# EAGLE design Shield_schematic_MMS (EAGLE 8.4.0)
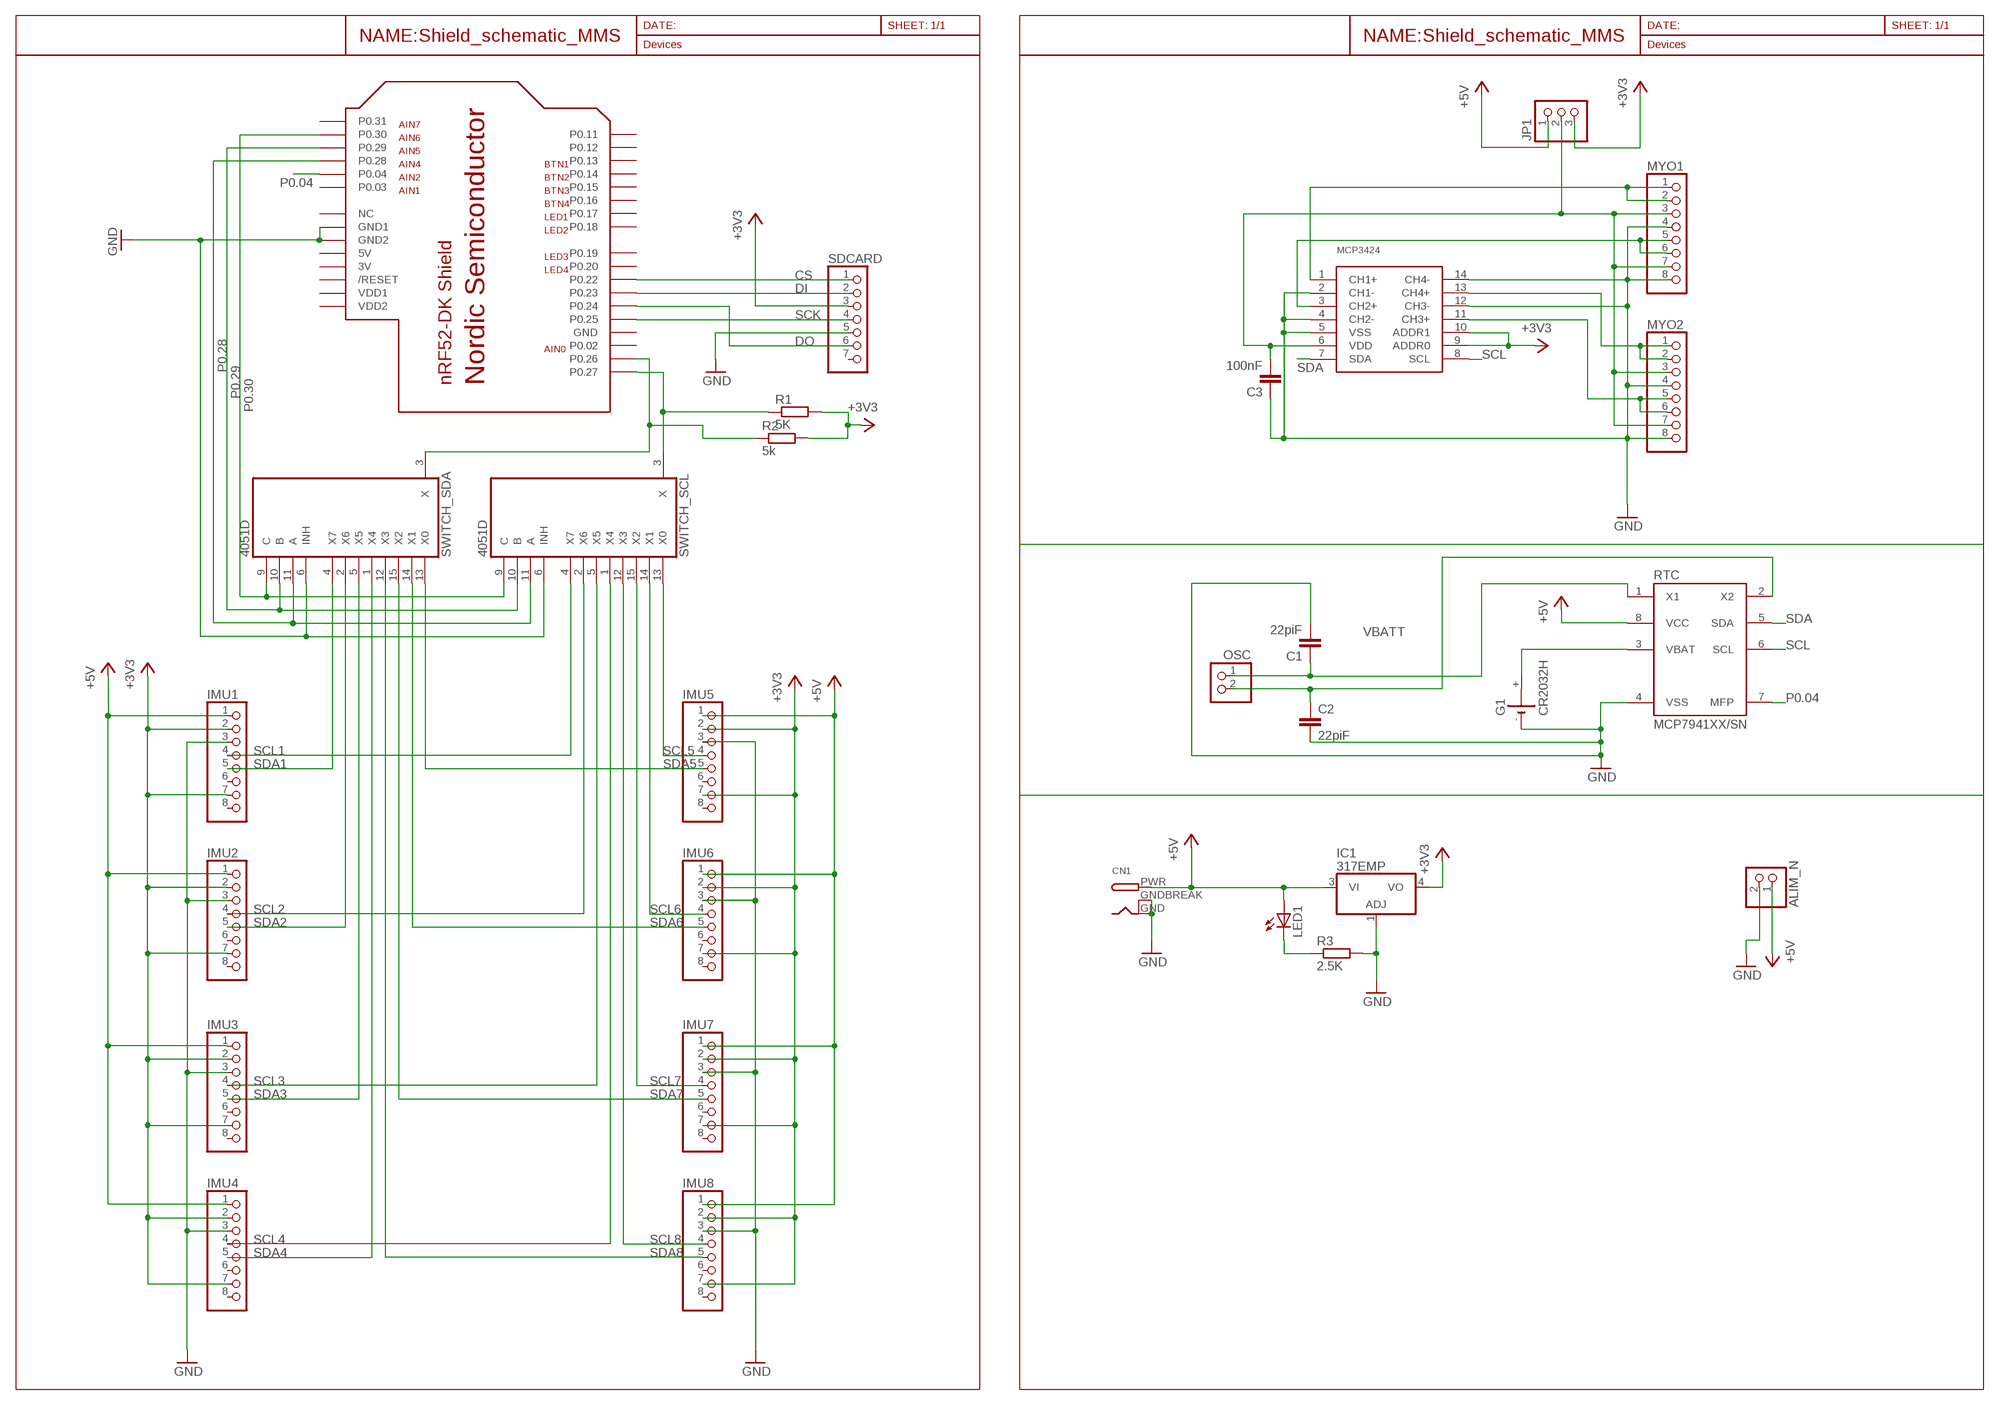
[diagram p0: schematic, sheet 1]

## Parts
ALIM_N  PINHD-1X2  [1X02]
C1  22piF  C2.5/2  [C2.5-2]
C2  22piF  C2.5/2  [C2.5-2]
C3  100nF  C2.5/2  [C2.5-2]
CN1  DCBARRELPTH  [DCJACK_2MM_PTH]
G1  CR2032H  [CR2032H]
IC1  317EMP  [SOT223]
IMU1  PINHD-1X8  [1X08]
IMU2  PINHD-1X8  [1X08]
IMU3  PINHD-1X8  [1X08]
IMU4  PINHD-1X8  [1X08]
IMU5  PINHD-1X8  [1X08]
IMU6  PINHD-1X8  [1X08]
IMU7  PINHD-1X8  [1X08]
IMU8  PINHD-1X8  [1X08]
JP1  PINHD-1X3  [1X03]
LED1  LEDCHIPLED_1206  [CHIPLED_1206]
MYO1  PINHD-1X8  [1X08]
MYO2  PINHD-1X8  [1X08]
OSC  PINHD-1X2  [1X02]
R1  5K  R-EU_M1206  [M1206]
R2  5k  R-EU_M1206  [M1206]
R3  2.5K  R-EU_M1206  [M1206]
RTC  MCP7941XX/SN  [SO8]
SDCARD  PINHD-1X7  [1X07]
SWITCH_SCL  4051D  [SO16]
SWITCH_SDA  4051D  [SO16]
U$2  NRF52-SHIELD-NOTEXT  [NRF52-SHIELD]
U$3  MCP3424  [SO14]

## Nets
+3V3: IC1.4(VO) IMU1.2 IMU1.7 IMU2.2 IMU2.7 IMU3.2 IMU3.7 IMU4.2 IMU4.7 IMU5.2 IMU5.7 IMU6.2 IMU6.7 IMU7.2 IMU7.7 IMU8.2 IMU8.7 JP1.3 R1.2 R2.2 SDCARD.3 U$3.9(ADDR0) U$3.10(ADDR1)
+5V: ALIM_N.1 CN1.PWR IC1.3(VI) IMU1.1 IMU2.1 IMU3.1 IMU4.1 IMU5.1 IMU6.1 IMU7.1 IMU8.1 JP1.1 LED1.A RTC.8(VCC)
CH1: MYO1.1 MYO1.2 U$3.1(CH1+)
CH2: MYO1.5 MYO1.6 U$3.3(CH2+)
CH3: MYO2.5 MYO2.6 U$3.11(CH3+)
CH4: MYO2.1 MYO2.2 U$3.13(CH4+)
CS: SDCARD.1 U$2.P22(P0.22)
DI: SDCARD.2 U$2.P23(P0.23)
DO: SDCARD.6 U$2.P24(P0.24)
GND: ALIM_N.2 C1.2 C2.2 C3.1 CN1.GND CN1.GNDBREAK G1.- IC1.1(ADJ) IMU1.3 IMU2.3 IMU3.3 IMU4.3 IMU5.3 IMU6.3 IMU7.3 IMU8.3 MYO1.4 MYO1.8 MYO2.4 MYO2.8 R3.2 RTC.4(VSS) SDCARD.5 SWITCH_SCL.6(INH) SWITCH_SDA.6(INH) U$2.GND1 U$2.GND2 U$3.2(CH1-) U$3.4(CH2-) U$3.5(VSS) U$3.12(CH3-) U$3.14(CH4-)
N$12: LED1.C R3.1
P0.04: RTC.7(MFP) U$2.P04(P0.04)
P0.28: SWITCH_SCL.11(A) SWITCH_SDA.11(A) U$2.P28(P0.28)
P0.29: SWITCH_SCL.10(B) SWITCH_SDA.10(B) U$2.P29(P0.29)
P0.30: SWITCH_SCL.9(C) SWITCH_SDA.9(C) U$2.P30(P0.30)
SCK: SDCARD.4 U$2.P25(P0.25)
SCL: R1.1 RTC.6(SCL) SWITCH_SCL.3(X) U$2.P27(P0.27) U$3.8(SCL)
SCL1: IMU1.4 SWITCH_SCL.4(X7)
SCL2: IMU2.4 SWITCH_SCL.2(X6)
SCL3: IMU3.4 SWITCH_SCL.5(X5)
SCL4: IMU4.4 SWITCH_SCL.1(X4)
SCL5: IMU5.4 SWITCH_SCL.13(X0)
SCL6: IMU6.4 SWITCH_SCL.14(X1)
SCL7: IMU7.4 SWITCH_SCL.15(X2)
SCL8: IMU8.4 SWITCH_SCL.12(X3)
SDA: R2.1 RTC.5(SDA) SWITCH_SDA.3(X) U$2.P26(P0.26) U$3.7(SDA)
SDA1: IMU1.5 SWITCH_SDA.4(X7)
SDA2: IMU2.5 SWITCH_SDA.2(X6)
SDA3: IMU3.5 SWITCH_SDA.5(X5)
SDA4: IMU4.5 SWITCH_SDA.1(X4)
SDA5: IMU5.5 SWITCH_SDA.13(X0)
SDA6: IMU6.5 SWITCH_SDA.14(X1)
SDA7: IMU7.5 SWITCH_SDA.15(X2)
SDA8: IMU8.5 SWITCH_SDA.12(X3)
VBATT: G1.+ RTC.3(VBAT)
VDD: C3.2 JP1.2 MYO1.3 MYO1.7 MYO2.3 MYO2.7 U$3.6(VDD)
X1: C1.1 OSC.1 RTC.1(X1)
X2: C2.1 OSC.2 RTC.2(X2)
Unconnected: G1.+@1(+) IMU1.6 IMU1.8 IMU2.6 IMU2.8 IMU3.6 IMU3.8 IMU4.6 IMU4.8 IMU5.6 IMU5.8 IMU6.6 IMU6.8 IMU7.6 IMU7.8 IMU8.6 IMU8.8 SDCARD.7 U$2.NC U$2.P02(P0.02) U$2.P03(P0.03) U$2.P11(P0.11) U$2.P12(P0.12) U$2.P13(P0.13) U$2.P14(P0.14) U$2.P15(P0.15) U$2.P16(P0.16) U$2.P17(P0.17) U$2.P18(P0.18) U$2.P19(P0.19) U$2.P20(P0.20) U$2.P31(P0.31) U$2.RESET(/RESET)

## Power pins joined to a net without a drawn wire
3V: U$2.3V
5V: U$2.5V
GND: SWITCH_SCL.8(GND) SWITCH_SDA.8(GND) U$2.GND
VCC: SWITCH_SCL.16(VCC) SWITCH_SDA.16(VCC)
VDD1: U$2.VDD2(VDD1)
VDD2: U$2.VDD1(VDD2)
VEE: SWITCH_SCL.7(VEE) SWITCH_SDA.7(VEE)

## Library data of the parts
ALIM_N OSC = pinhead:PINHD-1X2: PIN HEADER
C1-C3 = capacitor-wima:C: CAPACITOR
CN1 = adafruit:DCBARREL: 2.0mm DC Barrel Jack DCJACK_2MM_PTH - Through Hole Jack (4UConnector: 05537)
G1 = battery:CR2032H: LI BATTERY Varta
IC1 = linear:*317: Positive VOLTAGE REGULATOR
IMU1-IMU8 MYO1 MYO2 = pinhead:PINHD-1X8: PIN HEADER
JP1 = pinhead:PINHD-1X3: PIN HEADER
LED1 = adafruit:LED: LED
R1-R3 = resistor:R-EU_: RESISTOR, European symbol
RTC = _hhn_MCP7941X:MCP7941*?: Microchip MCP79410 / MCP79411 / MCP79412 I²C Real Time CLock/Calendar with Unique ID Rev. 5.0.0 as of 2013-10-23, for EAGLE 5+ Changelog 5.0.0 (initial) MCP79410XI/YY X: Unique ID 0: blank 1: EUI-48 2: EUI-96 I: Temperature Range (Industrial) /YY: Package /MS: MSOP8_.65 (8-Lead Micro Small Outline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
SDCARD = pinhead:PINHD-1X7: PIN HEADER
SWITCH_SCL SWITCH_SDA = 40xx:4051: 8-channel ANALOG MULTIPLEXER
U$2 = nrf52-shield_modif:NRF52-SHIELD: nRF5 devkit shield
U$3 = mcp3424:MCP3424

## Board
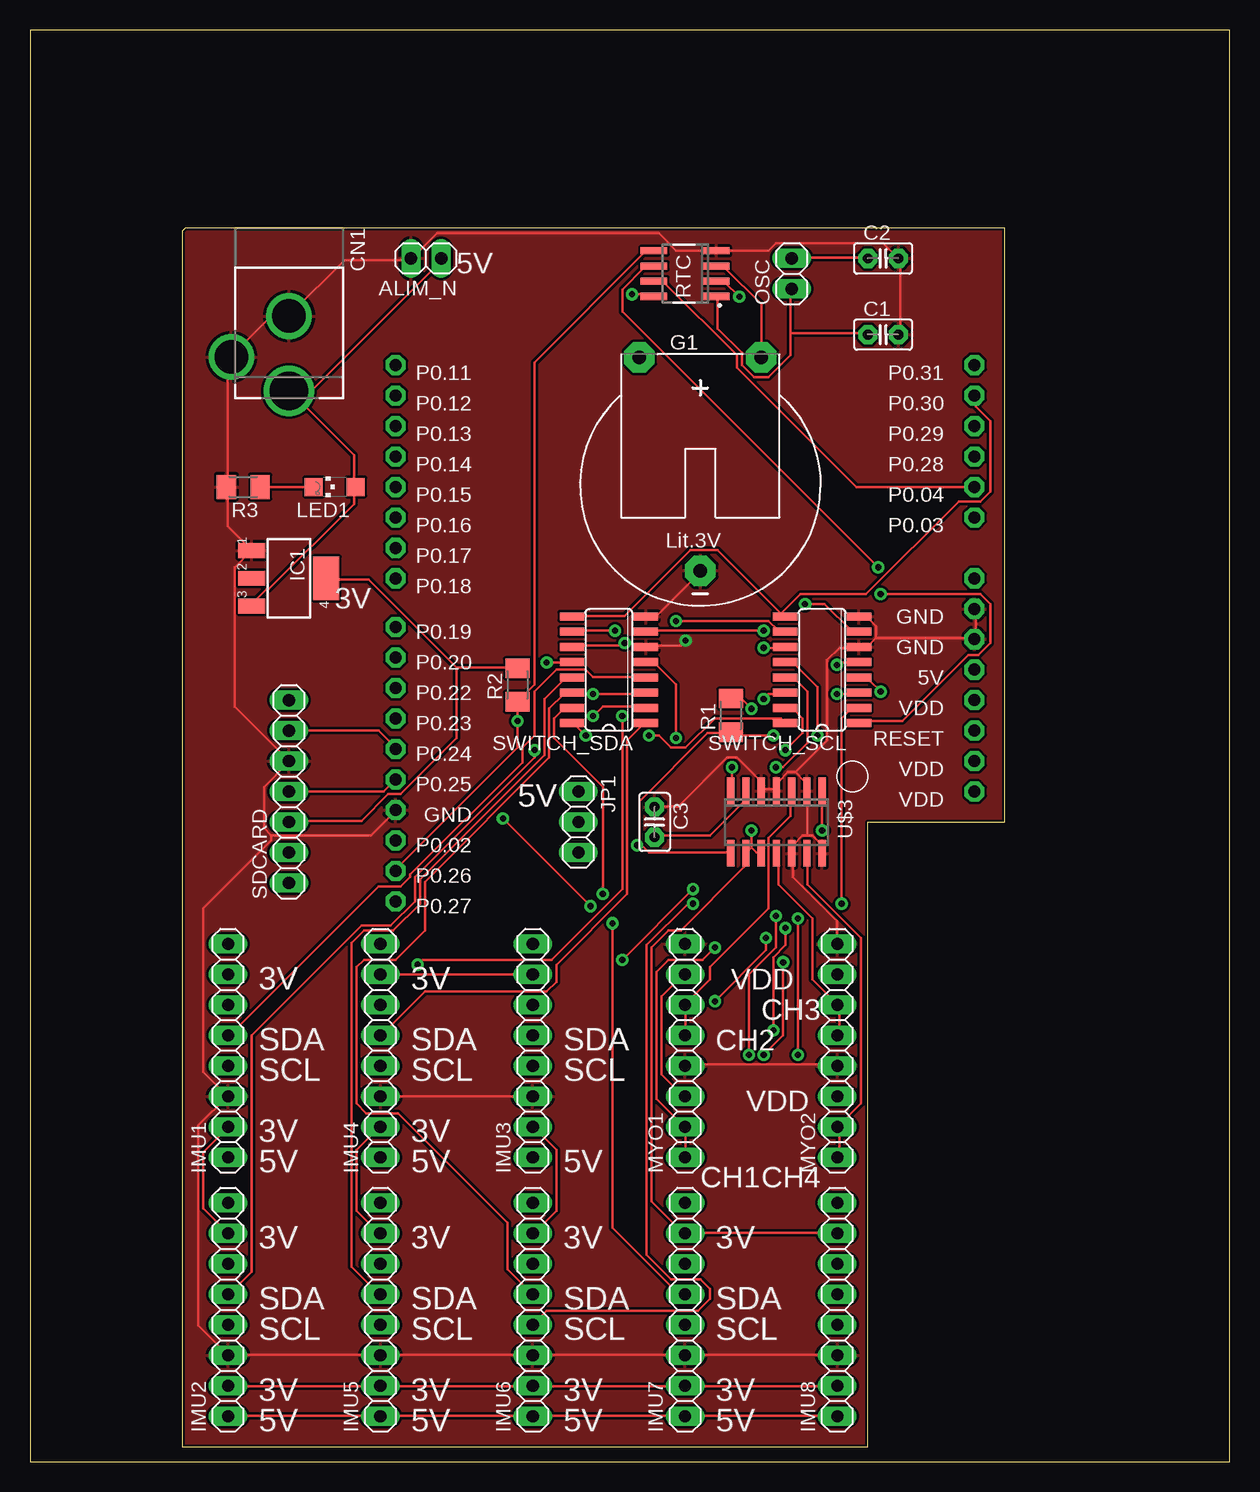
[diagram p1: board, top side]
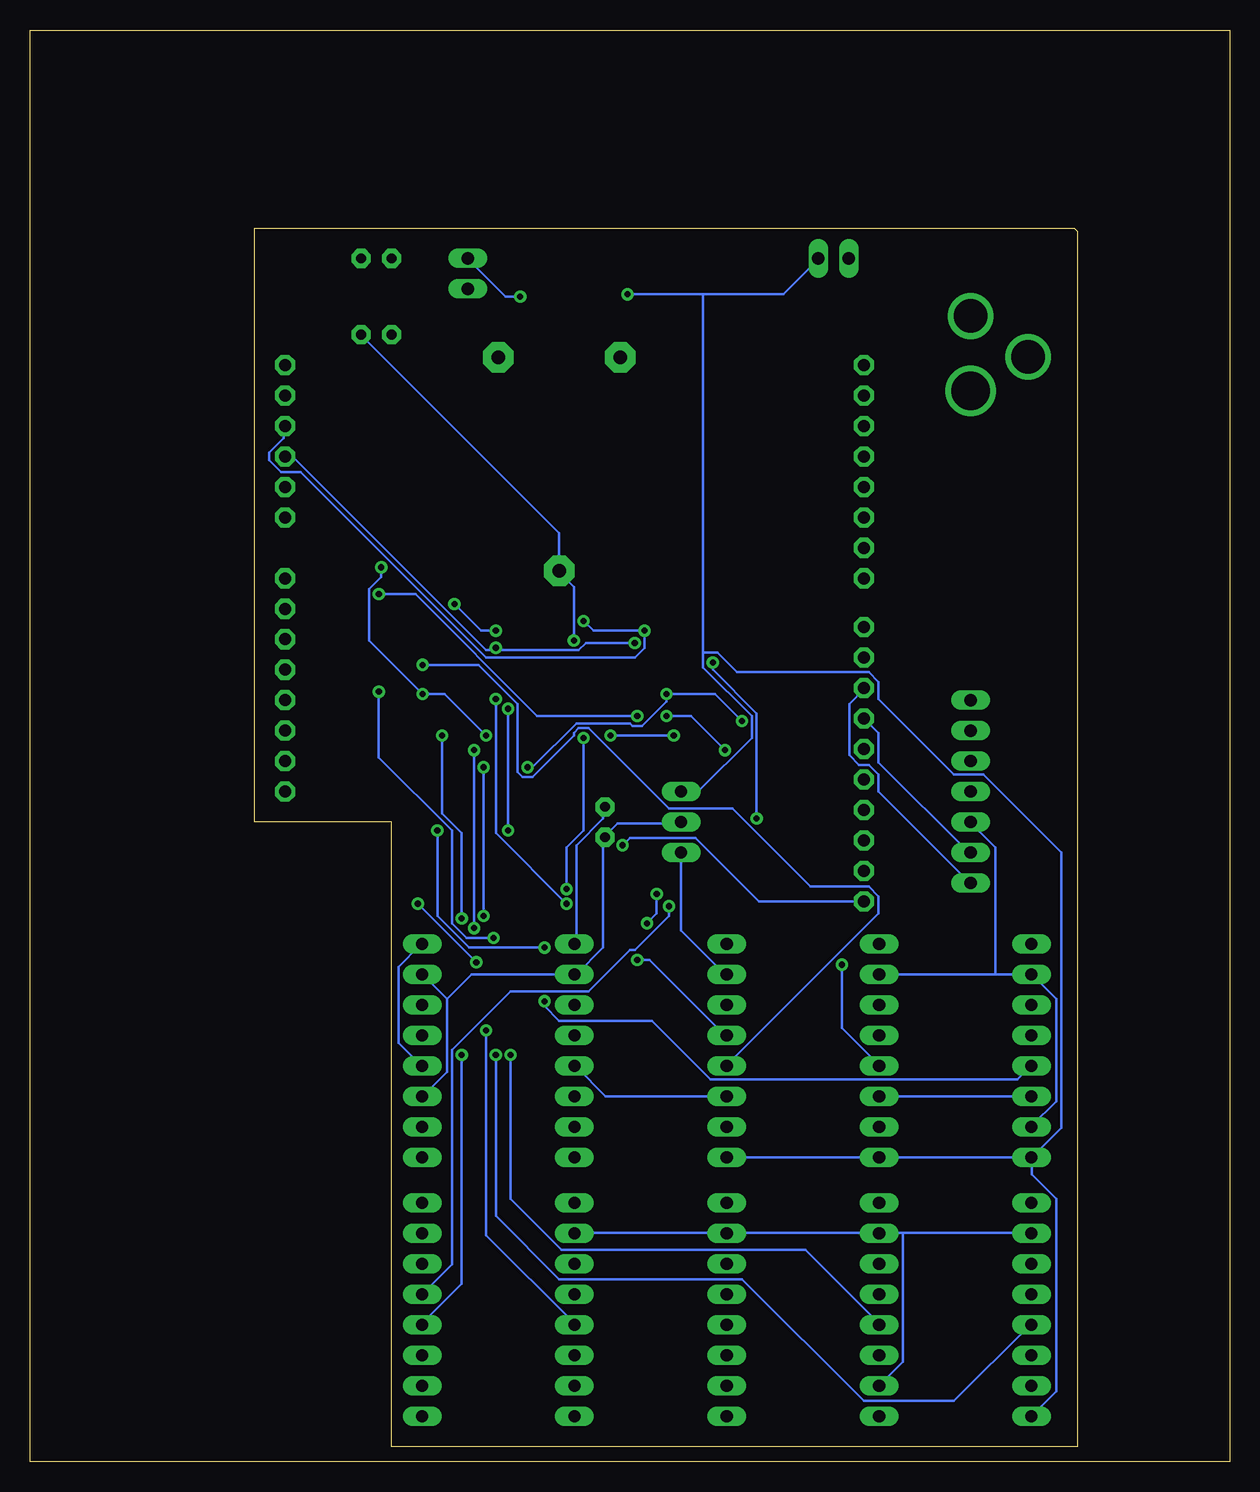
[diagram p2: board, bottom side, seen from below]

Size 100 x 119.37 mm. Coordinates in mm from the lower left corner, seen from the top.
Outline: 0,0 100,0 100,119.37 0,119.37 0,0
Copper layers (1*16): Top 0.035mm / dielectric 1.5mm / Bottom 0.035mm
Design rules "SparkFun": minimum track width 8mil, minimum drill 20mil, track to track 8mil, track to pad 8mil, pad to pad 8mil, via to via 8mil, smd to smd 8mil, copper to edge 8mil, drill to drill 8mil, minimum pad ring 12mil, minimum via ring 10mil, stop-mask expansion 4mil, vias tented up to drill 20mil, thermal gap 10mil

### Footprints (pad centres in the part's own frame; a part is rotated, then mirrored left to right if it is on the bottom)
1X02 = drill 1.016 long: 1 -1.27,0; 2 1.27,0
C2.5-2 = drill 0.813 pad 1.6 octagon: 1 -1.27,0; 2 1.27,0
DCJACK_2MM_PTH = drill 2.8: GND 0,7.35; GNDBREAK 4.8,10.75 | drill 3.2: PWR 0,13.6
CR2032H = drill 1.118 pad 2.54 octagon: + 5.08,10.795; +@1 -5.08,10.795; - 0,-6.985
SOT223 = smd 1.219 x 2.235: 1 -2.311,-3.099; 2 0,-3.099; 3 2.311,-3.099 | smd 3.6 x 2.2: 4 0,3.099
1X08 = drill 1.016 long: 1 -8.89,0; 2 -6.35,0; 3 -3.81,0; 4 -1.27,0; 5 1.27,0; 6 3.81,0; 7 6.35,0; 8 8.89,0
1X03 = drill 1.016 long: 1 -2.54,0; 2 0,0; 3 2.54,0
CHIPLED_1206 = smd 1.5 x 1.5: A 0,-1.75; C 0,1.75
M1206 = smd 1.6 x 2: 1 -1.4,0; 2 1.4,0
SO8 = smd 0.6 x 2.2: 1 -1.905,-2.6; 2 -0.635,-2.6; 3 0.635,-2.6; 4 1.905,-2.6; 5 1.905,2.6; 6 0.635,2.6; 7 -0.635,2.6; 8 -1.905,2.6
1X07 = drill 1.016 long: 1 -7.62,0; 2 -5.08,0; 3 -2.54,0; 4 0,0; 5 2.54,0; 6 5.08,0; 7 7.62,0
SO16 = smd 0.66 x 2.032: 1 -4.445,-3.073; 2 -3.175,-3.073; 3 -1.905,-3.073; 4 -0.635,-3.073; 5 0.635,-3.073; 6 1.905,-3.073; 7 3.175,-3.073; 8 4.445,-3.073; 9 4.445,3.073; 10 3.175,3.073; 11 1.905,3.073; 12 0.635,3.073; 13 -0.635,3.073; 14 -1.905,3.073; 15 -3.175,3.073; 16 -4.445,3.073
NRF52-SHIELD = drill 1 pad 1.676 octagon: 3V 62.23,1.27; 5V 64.77,1.27; GND 53.086,49.53; GND1 69.85,1.27; GND2 67.31,1.27; NC 72.39,1.27; P02 50.546,49.53; P03 77.47,1.27; P04 80.01,1.27; P11 90.17,49.53; P12 87.63,49.53; P13 85.09,49.53; P14 82.55,49.53; P15 80.01,49.53; P16 77.47,49.53; P17 74.93,49.53; P18 72.39,49.53; P19 68.326,49.53; P20 65.786,49.53; P22 63.246,49.53; P23 60.706,49.53; P24 58.166,49.53; P25 55.626,49.53; P26 48.006,49.53; P27 45.466,49.53; P28 82.55,1.27; P29 85.09,1.27; P30 87.63,1.27; P31 90.17,1.27; RESET 59.69,1.27; VDD1 57.15,1.27; VDD2 54.61,1.27
SO14 = smd 0.6 x 2.2: 1 -3.81,-2.6; 2 -2.54,-2.6; 3 -1.27,-2.6; 4 0,-2.6; 5 1.27,-2.6; 6 2.54,-2.6; 7 3.81,-2.6; 8 3.81,2.6; 9 2.54,2.6; 10 1.27,2.6; 11 0,2.6; 12 -1.27,2.6; 13 -2.54,2.6; 14 -3.81,2.6

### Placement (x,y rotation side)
ALIM_N  33.02,100.33 180 top
C1  71.12,93.98 0 top
C2  71.12,100.33 0 top
C3  52.07,53.34 270 top
CN1  21.59,102.87 180 top
G1  55.88,81.28 0 top
IC1  21.59,73.66 270 top
IMU1  16.51,34.29 90 top
IMU2  16.51,12.7 90 top
IMU3  41.91,34.29 90 top
IMU4  29.21,34.29 90 top
IMU5  29.21,12.7 90 top
IMU6  41.91,12.7 90 top
IMU7  54.61,12.7 90 top
IMU8  67.31,12.7 90 top
JP1  45.72,53.34 270 top
LED1  25.4,81.28 90 top
MYO1  54.61,34.29 90 top
MYO2  67.31,34.29 90 top
OSC  63.5,99.06 90 top
R1  58.42,62.23 90 top
R2  40.64,64.77 90 top
R3  17.78,81.28 180 top
RTC  54.61,99.06 90 top
SDCARD  21.59,55.88 90 top
SWITCH_SCL  66.04,66.04 90 top
SWITCH_SDA  48.26,66.04 90 top
U$2  80.01,1.27 90 top
U$3  62.23,53.34 180 top

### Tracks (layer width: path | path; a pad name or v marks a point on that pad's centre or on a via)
+3V3  (via drill 0.51)
  Top 0.203: 35.56,66.24 40.64,66.24 R2.2 | 35.56,66.24 28.25,73.56 24.79,73.56 IC1.4 | IMU4.7 IMU3.7 | 35.56,66.24 35.56,60.35 30.89,55.68 29.87,55.68 27.64,53.44 21.74,53.44 SDCARD.3 | IMU2.2 16.66,6.3 29.06,6.3 IMU5.2 29.26,6.3 41.86,6.3 IMU6.2 42.06,6.3 54.46,6.3 IMU7.2 54.66,6.3 67.26,6.3 IMU8.2 | IMU2.7 14.43,21.13 14.43,25.81 16.46,27.84 IMU1.2 | IMU5.7 29.06,19.1 27.23,20.93 27.23,26.01 29.06,27.84 IMU4.2 | v60.15,62.79 59.33,63.6 58.52,63.6 R1.2 | 60.15,51.21 v60.15,52.63 | 60.15,51.21 59.74,50.8 U$3.9 59.54,50.6 59.54,49.58 54.25,44.3 53.24,44.3 51.82,42.88 51.82,21.74 54.46,19.1 IMU7.7 54.66,19.1 67.26,19.1 IMU8.7 | 60.15,51.21 60.55,50.8 60.96,50.8 U$3.10 | IMU6.7 42.06,19.1 43.89,20.93 43.89,26.01 42.06,27.84 IMU3.2
  Bottom 0.203: JP1.3 45.72,44.3 42.06,40.64 IMU3.7 | IMU4.7 19.51,40.64 | 19.51,40.64 IMU1.7 16.46,40.64 14.43,38.61 14.43,30.07 16.46,28.04 IMU1.2 | 19.51,40.64 19.51,51.21 21.54,53.24 SDCARD.3 | 27.23,19.1 29.06,19.1 IMU5.7 29.26,19.1 41.86,19.1 IMU6.7 42.06,19.1 54.46,19.1 IMU7.7 | 27.23,19.1 16.66,19.1 IMU2.7 | v60.15,52.63 v60.15,62.79 | IMU5.2 27.23,8.33 27.23,19.1
+5V  (via drill 0.51)
  Top 0.203: IMU2.1 16.66,3.86 29.06,3.86 IMU5.1 29.26,3.86 41.86,3.86 IMU6.1 42.06,3.86 54.46,3.86 IMU7.1 54.66,3.86 67.26,3.86 IMU8.1 | 27.03,81.28 27.03,83.92 22.55,88.39 | 22.55,88.39 21.74,89.2 CN1.PWR 22.55,88.39 | 27.03,81.28 27.03,79.86 19.91,72.75 19.71,72.75 18.49,71.53 IC1.3 | 27.03,81.28 LED1.A | v50.19,97.33 51.82,97.33 RTC.8 | 22.55,88.39 34.34,100.18 ALIM_N.1
  Bottom 0.203: IMU3.1 IMU4.1 IMU1.1 16.46,25.4 | 16.46,25.4 16.46,23.98 14.43,21.95 14.43,5.89 IMU2.1 | 43.89,97.33 37.19,97.33 34.34,100.18 ALIM_N.1 | 43.89,97.33 v50.19,97.33 | JP1.1 44.3,55.88 39.83,60.35 39.83,62.18 43.89,66.24 43.89,67.46 | 43.89,97.33 43.89,67.46 | 16.46,25.4 14.02,27.84 14.02,50.8 20.52,57.3 22.96,57.3 29.26,63.6 29.26,65.02 30.07,65.84 41.05,65.84 42.67,67.46 43.89,67.46
CH1  (via drill 0.51)
  Top 0.203: v66.04,52.63 U$3.1 | v57.1,42.88 56.08,41.86 53.24,41.86 52.22,40.84 52.22,30.28 54.46,28.04 MYO1.2 54.66,27.84 54.66,25.4 MYO1.1
  Bottom 0.203: v66.04,52.63 66.04,45.52 63.4,42.88 v57.1,42.88
CH2
  Top 0.203: U$3.3 63.4,55.88 63.4,53.85 61.57,52.02 61.57,46.13 56.69,41.25 56.69,40.23 54.66,38.2 MYO1.6 54.66,38 54.66,35.56 MYO1.5
CH3
  Top 0.203: U$3.11 62.38,50.6 62.38,48.16 65.23,45.31 65.23,40.23 67.26,38.2 MYO2.6 67.46,38 67.46,35.56 MYO2.5
CH4
  Top 0.203: U$3.13 64.82,50.6 64.82,48.16 69.29,43.69 69.29,29.87 67.46,28.04 MYO2.2 67.46,27.84 67.46,25.4 MYO2.1
CS
  Bottom 0.203: SDCARD.1 21.74,48.36 29.26,55.88 29.26,57.3 30.07,58.12 30.89,58.12 31.7,58.93 31.7,63.2 30.48,64.41 U$2.P22
DI
  Bottom 0.203: U$2.P23 29.26,60.76 29.26,58.32 21.74,50.8 SDCARD.2
DO
  Top 0.203: SDCARD.6 29.06,60.96 30.48,59.54 U$2.P24
GND  (via drill 0.51)
  Top 0.203: v54.66,68.48 54.25,68.07 51.41,68.07 SWITCH_SDA.6 | SWITCH_SDA.8 51.41,70.51 52.22,70.51 55.88,74.17 G1.- | C1.2 72.54,94.08 72.54,100.18 C2.2 71.12,101.6 62.18,101.6 61.57,100.99 57.3,100.99 RTC.4 57.1,100.99 53.85,100.99 52.43,102.41 33.93,102.41 31.9,100.38 ALIM_N.2 31.7,100.18 26.21,100.18 21.74,95.71 CN1.GND 21.54,95.5 20.12,95.5 16.87,92.25 CN1.GNDBREAK 16.66,92.05 16.46,91.85 16.46,81.28 | 20.12,52.22 19.51,52.83 19.51,56.29 21.54,58.32 SDCARD.5 21.54,58.52 17.07,62.99 17.07,74.57 18.49,76 | 20.12,52.22 28.45,52.22 30.48,54.25 U$2.GND | 16.46,81.28 16.46,78.03 18.49,76 | 16.46,81.28 R3.2 | 18.49,76 IC1.1 | IMU8.3 67.26,8.94 54.66,8.94 IMU7.3 54.46,8.94 42.06,8.94 IMU6.3 41.86,8.94 29.26,8.94 IMU5.3 29.06,8.94 16.66,8.94 IMU2.3 14.02,11.38 14.02,28.04 16.46,30.48 | IMU4.3 IMU3.3 | MYO1.4 54.66,33.12 67.26,33.12 MYO2.4 | 70.51,68.68 69.9,68.07 69.29,68.07 SWITCH_SCL.6 69.09,67.87 67.46,67.87 66.45,66.85 66.45,60.15 63.8,57.51 | 70.51,68.68 70.51,69.7 69.9,70.31 69.29,70.31 SWITCH_SCL.8 | 70.51,68.68 78.64,68.68 U$2.GND2 78.84,68.68 78.84,71.12 U$2.GND1 | 60.96,56.08 62.18,56.08 U$3.4 62.38,56.08 62.38,56.69 63.2,57.51 63.8,57.51 | 64.82,52.22 65.23,52.22 66.04,51.41 U$3.14 | 64.82,52.22 64.41,52.22 63.6,51.41 63.6,50.8 U$3.12 63.6,50.6 63.6,48.77 67.26,45.11 67.26,43.28 MYO2.8 | 64.82,52.22 64.82,55.88 U$3.2 64.62,56.08 64.62,56.69 63.8,57.51 | 60.96,56.08 60.96,56.69 58.93,58.73 58.12,58.73 54.05,54.66 52.22,54.66 C3.1 | 60.96,56.08 U$3.5 | 20.12,52.22 20.12,51.82 14.43,46.13 14.43,32.51 16.46,30.48 | 16.46,30.48 IMU1.3
  Bottom 0.203: v54.66,68.48 54.66,72.95 55.88,74.17 G1.- 55.88,77.42 72.34,93.88 C1.2 | IMU4.3 IMU1.3 | C3.1 52.22,54.46 52.22,53.65 54.46,51.41 54.46,43.28 MYO1.8 | MYO2.4 67.46,33.12 69.29,34.95 69.29,41.25 67.46,43.08 MYO2.8 | IMU3.3 52.02,30.48 54.46,32.92 MYO1.4
  pour Top: 12.7,102.87 81.28,102.87 81.28,53.34 69.85,53.34 69.85,1.27 12.7,1.27
N$12
  Top 0.203: R3.1 LED1.C
P0.04
  Top 0.203: U$2.P04 68.89,81.28 58.93,91.24 58.93,92.25 52.83,98.35 52.02,98.35 RTC.7
P0.28  (via drill 0.51)
  Top 0.203: v49.58,68.28 49.38,68.07 45.31,68.07 SWITCH_SDA.11 | v61.16,67.87 62.79,67.87 SWITCH_SCL.11
  Bottom 0.203: v49.58,68.28 53.65,68.28 54.25,67.67 61.16,67.67 | 61.16,67.67 61.98,67.67 78.03,83.72 78.64,83.72 U$2.P28 | 61.16,67.67 v61.16,67.87
P0.29  (via drill 0.51)
  Top 0.203: v48.77,69.29 45.31,69.29 SWITCH_SDA.10 | v53.85,70.1 61.57,70.1 62.38,69.29 62.79,69.29 SWITCH_SCL.10
  Bottom 0.203: v53.85,70.1 53.03,69.29 v48.77,69.29 48.77,67.87 49.58,67.06 61.98,67.06 77.42,82.5 79.05,82.5 80.06,83.52 80.06,84.12 78.84,85.34 78.84,86.36 U$2.P29
P0.30
  Top 0.203: 62.59,70.71 62.79,70.51 SWITCH_SCL.9 62.59,70.71 | 62.59,70.71 57.3,76 55.07,76 49.58,70.51 45.31,70.51 SWITCH_SDA.9 | 62.59,70.71 64.21,72.34 69.7,72.34 77.42,80.06 79.25,80.06 80.06,80.87 80.06,86.77 78.84,87.99 78.84,88.8 U$2.P30
SCK
  Top 0.203: SDCARD.4 29.46,55.88 U$2.P25
SCL  (via drill 0.51)
  Top 0.203: 50.8,51.61 50.8,55.07 56.49,60.76 58.32,60.76 R1.1 58.52,60.76 58.73,60.55 v61.98,60.55 | 50.8,51.61 51.61,50.8 58.32,50.8 U$3.8 | v67.26,64.01 69.09,64.01 SWITCH_SCL.3 | v70.71,74.57 49.38,95.91 49.38,97.74 51.21,99.57 51.82,99.57 RTC.6 | 50.8,51.61 v50.6,51.41
  Bottom 0.203: v61.98,60.55 65.43,64.01 v67.26,64.01 71.73,68.48 71.73,72.75 70.71,73.76 v70.71,74.57 | U$2.P27 39.22,46.74 44.5,52.02 49.99,52.02 v50.6,51.41
SCL1  (via drill 0.51)
  Top 0.203: v70.92,64.21 69.9,65.23 69.29,65.23 SWITCH_SCL.4 | v61.37,43.69 61.37,42.67 v57.1,38.41
  Bottom 0.203: v70.92,64.21 70.92,58.73 64.82,52.63 64.82,44.91 63.6,43.69 v61.37,43.69 | v57.1,38.41 57.1,38 55.88,36.78 48.16,36.78 43.28,31.9 17.68,31.9 16.66,32.92 IMU1.4
SCL2  (via drill 0.51)
  Top 0.203: v67.67,46.53 67.67,61.98 68.48,62.79 69.09,62.79 SWITCH_SCL.2 | v62.79,41.66 62.79,35.56 v61.16,33.93
  Bottom 0.203: v62.79,41.66 v67.67,46.53 | v61.16,33.93 61.16,20.52 55.88,15.24 40.64,15.24 30.48,5.08 22.96,5.08 16.66,11.38 IMU2.4
SCL3  (via drill 0.51)
  Top 0.203: v67.26,66.45 67.46,66.65 69.09,66.65 SWITCH_SCL.5
  Bottom 0.203: v67.26,66.45 62.59,66.45 59.33,63.2 59.33,57.51 58.93,57.1 58.12,57.1 54.66,60.55 54.66,60.76 54.25,61.16 53.44,61.16 46.74,54.46 41.45,54.46 34.95,47.95 30.07,47.95 29.26,47.14 29.26,45.72 41.86,33.12 IMU3.4
SCL4  (via drill 0.51)
  Top 0.203: v70.92,72.34 79.25,72.34 80.06,71.53 80.06,68.28 79.05,67.26 78.23,67.26 72.75,61.77 69.29,61.77 SWITCH_SCL.1 | v49.38,62.18 49.38,47.75 43.48,41.86 32.72,41.86 v32.31,41.45
  Bottom 0.203: v70.92,72.34 67.87,72.34 57.71,62.18 v49.38,62.18 | v32.31,41.45 32.31,36.17 29.26,33.12 IMU4.4
SCL5  (via drill 0.51)
  Top 0.203: v62.18,57.91 62.79,57.91 64.82,59.94 64.82,64.21 63.8,65.23 62.99,65.23 SWITCH_SCL.13 | v62.18,45.52 62.18,42.88 59.94,40.64 v59.94,33.93
  Bottom 0.203: v62.18,45.52 v62.18,57.91 | v59.94,33.93 59.94,21.95 55.68,17.68 35.36,17.68 29.26,11.58 IMU5.4
SCL6  (via drill 0.51)
  Top 0.203: v61.16,63.6 61.57,64.01 62.79,64.01 SWITCH_SCL.14 | v55.27,46.53 54.86,46.53 51.41,43.08 51.41,17.27 53.44,15.24 55.88,15.24 56.69,14.43 56.69,13.61 55.68,12.6 43.08,12.6 IMU6.4
  Bottom 0.203: v61.16,63.6 61.16,52.43 v55.27,46.53
SCL7  (via drill 0.51)
  Top 0.203: v62.99,59.33 64.41,60.76 64.41,61.98 63.6,62.79 62.99,62.79 SWITCH_SCL.15 | v62.99,44.5 62.99,43.08 61.98,42.06 v61.98,35.97
  Bottom 0.203: v62.99,44.5 v62.99,59.33 | v61.98,35.97 61.98,18.9 54.66,11.58 IMU7.4
SCL8  (via drill 0.51)
  Top 0.203: v65.63,60.55 65.63,64.62 63.6,66.65 62.99,66.65 SWITCH_SCL.12 | v64.01,33.93 v64.01,45.31
  Bottom 0.203: v65.63,60.55 65.63,54.05 64.01,52.43 v64.01,45.31 | v64.01,33.93 64.01,14.83 67.26,11.58 IMU8.4
SDA  (via drill 0.51)
  Top 0.203: U$2.P26 30.48,49.38 40.64,59.54 v40.64,61.77 R2.1 40.64,63.4 42.06,64.82 42.06,91.64 51.21,100.79 51.82,100.79 RTC.5 | v46.94,64.01 51.21,64.01 SWITCH_SDA.3 | v58.52,57.91 58.52,56.08 U$3.7
  Bottom 0.203: v40.64,61.77 42.88,64.01 v46.94,64.01 46.94,63.4 48.97,61.37 49.78,61.37 49.99,61.57 54.46,61.57 58.12,57.91 v58.52,57.91
SDA1
  Top 0.203: SWITCH_SDA.4 51.21,65.43 46.94,65.43 46.33,66.04 43.89,66.04 42.06,64.21 42.06,60.55 41.05,59.54 41.05,58.32 31.7,48.97 31.7,48.77 30.89,47.95 29.06,47.95 16.66,35.56 IMU1.5
SDA2  (via drill 0.51)
  Top 0.203: v46.94,62.18 47.75,62.99 51.21,62.99 SWITCH_SDA.2 | v42.06,59.33 42.06,58.73 32.11,48.77 32.11,46.74 30.07,44.7 27.64,44.7 18.49,35.56 18.49,15.85 16.66,14.02 IMU2.5
  Bottom 0.203: v46.94,62.18 44.91,62.18 v42.06,59.33
SDA3  (via drill 0.51)
  Top 0.203: v53.85,60.35 53.85,64.82 52.02,66.65 51.41,66.65 SWITCH_SDA.5 | v49.38,41.86 v55.27,47.75
  Bottom 0.203: v53.85,60.35 53.85,52.63 55.27,51.21 v55.27,47.75 | v49.38,41.86 48.36,41.86 42.06,35.56 IMU3.5
SDA4
  Top 0.203: SWITCH_SDA.1 51.21,61.57 49.78,60.15 49.78,47.35 43.89,41.45 43.89,40.03 43.08,39.22 32.92,39.22 29.26,35.56 IMU4.5
SDA5
  Top 0.203: SWITCH_SDA.13 45.11,65.23 44.5,65.23 42.88,63.6 42.88,58.93 32.51,48.56 32.51,46.53 30.28,44.3 27.84,44.3 26.82,43.28 26.82,16.26 29.06,14.02 IMU5.5
SDA6
  Top 0.203: IMU6.5 39.83,16.05 39.83,19.91 30.68,29.06 28.04,29.06 27.23,29.87 27.23,41.25 27.84,41.86 30.48,41.86 32.92,44.3 32.92,48.36 43.28,58.73 43.28,62.79 44.5,64.01 45.11,64.01 SWITCH_SDA.14
SDA7  (via drill 0.51)
  Top 0.203: v47.75,47.35 47.75,56.29 43.69,60.35 43.69,61.98 44.5,62.79 45.11,62.79 SWITCH_SDA.15 | v48.56,44.91 48.56,19.51 54.05,14.02 54.46,14.02 IMU7.5
  Bottom 0.203: v47.75,47.35 47.75,45.72 v48.56,44.91
SDA8  (via drill 0.51)
  Top 0.203: v43.08,66.65 45.11,66.65 SWITCH_SDA.12 | v46.74,46.33 v39.42,53.65
  Bottom 0.203: v43.08,66.65 43.08,66.04 39.42,62.38 v39.42,53.65 | v46.74,46.33 46.74,45.52 49.58,42.67 49.99,42.67 53.44,39.22 59.94,39.22 64.82,34.34 64.82,16.46 IMU8.5
VBATT
  Top 0.203: G1.+ 60.96,96.52 57.91,99.57 57.3,99.57 RTC.3
VCC  (via drill 0.51)
  Top 0.203: v46.33,60.55 45.31,61.57 SWITCH_SDA.16 | v51.61,60.55 52.43,60.55 53.44,59.54 54.66,59.54 57.1,61.98 62.59,61.98 SWITCH_SCL.16
  Bottom 0.203: v51.61,60.55 v46.33,60.55
VDD
  Top 0.203: U$3.6 59.54,55.88 59.54,55.07 56.69,52.22 52.22,52.22 C3.2 | MYO1.3 54.46,30.48 52.63,32.31 52.63,38.81 54.46,40.64 MYO1.7
  Bottom 0.203: JP1.2 45.72,53.24 51,53.24 52.02,52.22 C3.2 52.22,52.02 52.22,42.88 54.46,40.64 MYO1.7 63.2,40.64 65.23,38.61 | 65.23,38.61 65.23,32.51 67.26,30.48 MYO2.3 | 65.23,38.61 67.26,40.64 MYO2.7
VEE  (via drill 0.51)
  Top 0.203: v61.16,69.29 51.41,69.29 SWITCH_SDA.7 | v64.62,71.53 66.24,71.53 68.48,69.29 69.09,69.29 SWITCH_SCL.7
  Bottom 0.203: v61.16,69.29 62.38,69.29 v64.62,71.53
X1
  Top 0.203: 63.4,94.08 63.4,97.74 OSC.1 | 63.4,94.08 63.4,92.25 61.57,90.42 60.35,90.42 59.33,91.44 59.33,92.46 57.3,94.49 57.3,97.13 RTC.1 | 63.4,94.08 69.7,94.08 C1.1
X2  (via drill 0.51)
  Top 0.203: v59.13,97.13 57.91,98.35 57.3,98.35 RTC.2 | C2.1 69.7,100.38 63.6,100.38 OSC.2
  Bottom 0.203: v59.13,97.13 60.35,97.13 63.4,100.18 OSC.2

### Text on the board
tPlace: 5V | 3V | 5V | 3V | 3V | VDD | CH3 | SDA | SDA | SDA | CH2 | SCL | SCL | SCL | VDD | 3V | 3V | 5V | 5V | 5V | CH1 | CH4 | 3V | 3V | 3V | 3V | SDA | SDA | SDA | SDA | SCL | SCL | SCL | SCL | 3V | 3V | 3V | 3V | 5V | 5V | 5V | 5V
